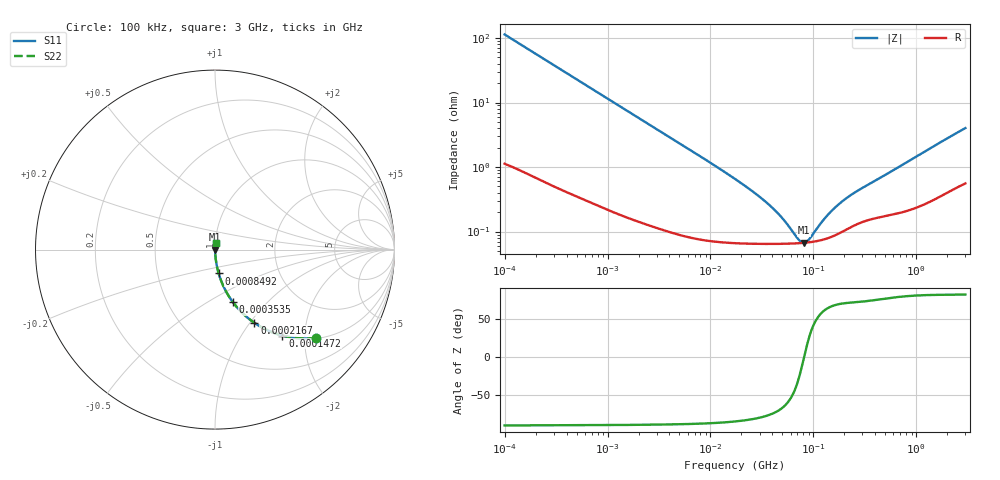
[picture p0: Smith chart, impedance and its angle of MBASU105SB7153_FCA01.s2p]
! MBASU105SB7153_FCA01  S-PARAMETER MODEL  ( Standard Model )
! Model Generated by TAIYO YUDEN Corporation (http://www.ty-top.com)
! Version 1.0
! TAIYO YUDEN Control No. 220601
! Copyright(c) 2021 TAIYO YUDEN CO.,LTD. All Rights Reserved.
! Product Description (link to TY-COMPAS)
! https://ds.yuden.co.jp/TYCOMPAS/or/detail?pn=MBASU105SB7153KFCA01&u=M
! Products Name : Multilayer Ceramic Capacitors
! Characteristics :
!  Capacitance : 0.015 [uF] , Rated Voltage : 50 [V] , TCC : X7R
!  Case Size : 1.0 x 0.5 / 0.039 x 0.02 [mm/inch] , Thickness : 0.5 / 0.02 [mm/inch]
!  (Conditions: Temperature = 25 [degC] , DC Bias Voltage = 0 [V])
! External Node Assignments :
!  1  o---| |---o  2
! GND o---------o GND
! Frequency Range : 100kHz  -  3GHz  [ 401 STEP ]
# MHZ S RI R 50
! Freq[MHz].  S11 Real  S11 Imag  S21 Real  S21 Imag  S12 Real  S12 Imag  S22 Real  S22 Imag
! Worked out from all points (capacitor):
!   401 points, 100 kHz to 3 GHz, reference 50 ohm
!   read as one part in series: C = 14 nF near 105.3 kHz
!   lowest |Z| = 66.9 mohm at 81.31 MHz (marker M1)
!   series resonance near 81.2 MHz, so ESL is about 270 pH
!   S11 on the Smith chart (normalised r, x): 100 kHz: 1.02, -2.27; 147.2 kHz: 1.02, -1.55; 216.7 kHz: 1.01, -1.05; 353.5 kHz: 1.01, -0.65; 849.2 kHz: 1.00, -0.27; 3 GHz: 1.01, +0.08
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0.1  0.5623 -0.4912  0.4377 0.4912  0.4377 0.4912  0.5623 -0.4912
0.147195  0.3755 -0.4787  0.6245 0.4787  0.6245 0.4787  0.3755 -0.4787
0.216663  0.22 -0.4082  0.78 0.4082  0.78 0.4082  0.22 -0.4082
0.353547  0.0982 -0.2908  0.9018 0.2908  0.9018 0.2908  0.0982 -0.2908
0.562235  0.043 -0.1951  0.957 0.1951  0.957 0.1951  0.043 -0.1951
0.849186  0.0204 -0.1328  0.9796 0.1328  0.9796 0.1328  0.0204 -0.1328
1.536162  0.00729 -0.0748  0.9927 0.0748  0.9927 0.0748  0.00729 -0.0748
3.161081  0.00246 -0.0368  0.9975 0.0368  0.9975 0.0368  0.00246 -0.0368
17.7727  0.000698 -0.00632  0.9993 0.00632  0.9993 0.00632  0.000698 -0.00632
27.54426  0.000659 -0.00379  0.9993 0.00379  0.9993 0.00379  0.000659 -0.00379
38.50681  0.000648 -0.00238  0.9994 0.00238  0.9994 0.00238  0.000648 -0.00238
51.12795  0.000648 -0.0014  0.9994 0.0014  0.9994 0.0014  0.000648 -0.0014
71.47675  0.000659 -0.000374  0.9993 0.000374  0.9993 0.000374  0.000659 -0.000374
77.22239  0.000664 -0.000147  0.9993 0.000147  0.9993 0.000147  0.000664 -0.000147
81.30716  0.000669 3.83e-06  0.9993 -3.83e-06  0.9993 -3.83e-06  0.000669 3.83e-06
87.84301  0.000677 0.000231  0.9993 -0.000231  0.9993 -0.000231  0.000677 0.000231
97.38194  0.000691 0.000536  0.9993 -0.000536  0.9993 -0.000536  0.000691 0.000536
132.6759  0.000773 0.0015  0.9992 -0.0015  0.9992 -0.0015  0.000773 0.0015
185.4806  0.000975 0.00266  0.999 -0.00266  0.999 -0.00266  0.000975 0.00266
259.3015  0.00129 0.00393  0.9987 -0.00393  0.9987 -0.00393  0.00129 0.00393
547.5153  0.00185 0.00799  0.9982 -0.00799  0.9982 -0.00799  0.00185 0.00799
3000  0.00711 0.0393  0.9929 -0.0393  0.9929 -0.0393  0.00711 0.0393
